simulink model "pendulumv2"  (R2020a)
settings: Solver=ode45  StartTime=0.0  StopTime=10  RelTol=1e-3  EnableMultiTasking=on
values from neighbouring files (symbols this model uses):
  q10 = pi*theta0/180    (= 2.09439510239)    [pendulumdemo.m]
  q1L0 = q10    (= 2.09439510239)    [pendulumdemo.m]
  q20 = 0    [pendulumdemo.m]
  q2L0 = 0    [pendulumdemo.m]

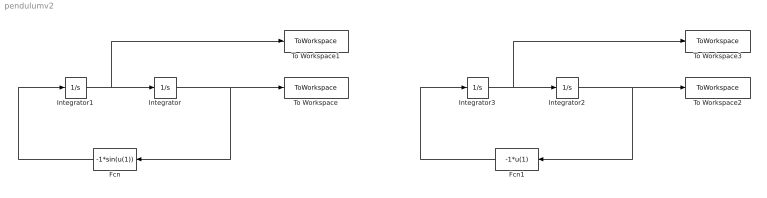
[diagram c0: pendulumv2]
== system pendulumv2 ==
  Fcn : Fcn  Expr=-1*sin(u(1))
  Fcn1 : Fcn  Expr=-1*u(1)
  Integrator : Integrator  InitialCondition=q10
  Integrator1 : Integrator  InitialCondition=q20
  Integrator2 : Integrator  InitialCondition=q1L0
  Integrator3 : Integrator  InitialCondition=q2L0
  To Workspace : ToWorkspace  VariableName=q1  SampleTime=-1
  To Workspace1 : ToWorkspace  VariableName=q2  SampleTime=-1
  To Workspace2 : ToWorkspace  VariableName=q1L  SampleTime=-1
  To Workspace3 : ToWorkspace  VariableName=q2L  SampleTime=-1
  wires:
  Fcn/1 -> Integrator1/1
  Integrator1/1 -> To Workspace1/1, Integrator/1
  Integrator/1 -> To Workspace/1, Fcn/1
  Integrator2/1 -> To Workspace2/1, Fcn1/1
  Integrator3/1 -> To Workspace3/1, Integrator2/1
  Fcn1/1 -> Integrator3/1
